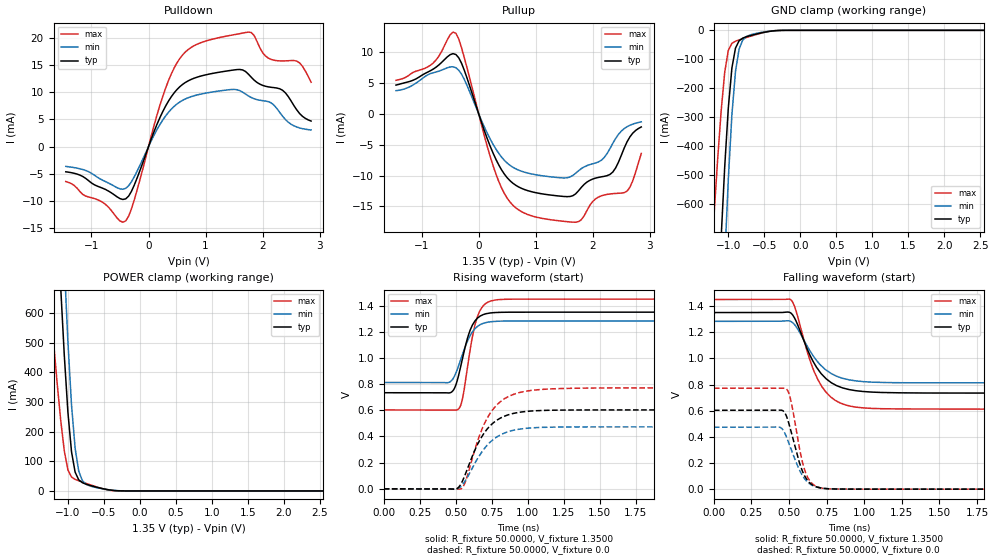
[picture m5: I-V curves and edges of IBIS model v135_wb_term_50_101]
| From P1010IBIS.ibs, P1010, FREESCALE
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[Model] v135_wb_term_50_101
|   Model v135_wb_term_50_101
| This model was characterised for following simulation conditions:
| External (pad) voltage:
|   - Typ: 1.35V,   - Min: 1.283V,   - Max: 1.45V
| Library cells for typ/min/max conditions are connected as defined below:
|  chip_pad - External Pad
|  ipp_do - Core Input
|  ipp_obe - Output Buffer Enable
|  esd_boost - vdd_io
|  gnd_io - gnd_io
|  vdd_d - vdd_d
|  vdd_io - vdd_io
|  vipp_dse_0 - gnd_io vdd_d gnd_io
|  vipp_dse_1 - vdd_d vdd_d gnd_io
|  vipp_dse_2 - vdd_d gnd_io gnd_io
|  vipp_dse_3 - gnd_io
|  vipp_dse_4 - gnd_io vdd_d gnd_io
|  vipp_dse_5 - vdd_d vdd_d gnd_io
|  vipp_dse_6 - vdd_d gnd_io vdd_d
|  vipp_dse_7 - gnd_io vdd_d gnd_io
|  vsel[0] - vdd_d
|  vsel[1] - gnd_io
|  vtermsel_0 - vdd_d
|  vtermsel_1 - gnd_io
|  vtermsel_2 - vdd_d
| All other pins connected to ground
Model_type I/O
Polarity   Non-Inverting
Enable   Active-High
Vinl =   0.5150V
Vinh =   0.9350V
Vmeas =  0.6750V
Cref =   0.0F
Rref =   50.0000
Vref =   0.6750V
C_comp   2.2026pF   1.9235pF   2.5884pF
[Receiver Thresholds]
Vth   =  0.675V
Vinh_ac  =  0.160V
Vinh_dc  =  0.090V
Vinl_ac  = -0.160V
Vinl_dc  = -0.090V
[Temperature Range]   65.0000   0.1250k   -40.0000
[Voltage Range]   1.3500V   1.2830V   1.4500V
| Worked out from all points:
|   slope of the pulldown table from 0 to 0.203 V, typ, clamps not added: 37.5 ohm
|   slope of the pullup table from 0 to 0.203 V, typ, clamps not added: 38.4 ohm
|   GND clamp passes 1 mA (typ) near -0.33 V on its own axis
|   POWER clamp passes 1 mA (typ) near -0.33 V on its own axis
|   rising waveform, R_fixture 50.0000, V_fixture 1.3500: 20-80 % time 87.9ps typ, 100ps min, 80.4ps max; typ from 0.734 V to 1.35 V
|   rising waveform, R_fixture 50.0000, V_fixture 0.0: 20-80 % time 169ps typ, 179ps min, 171ps max; typ from 0 V to 0.603 V
|   falling waveform, R_fixture 50.0000, V_fixture 1.3500: 20-80 % time 167ps typ, 176ps min, 157ps max; typ from 1.35 V to 0.734 V
|   falling waveform, R_fixture 50.0000, V_fixture 0.0: 20-80 % time 91.9ps typ, 104ps min, 79.1ps max; typ from 0.603 V to 0 V
[Pulldown]
|Voltage   I(typ)   I(min)   I(max)
-1.45V    -4.625mA   -3.634mA   -6.414mA
-400mV    -9.605mA   -7.673mA   -13.66mA
-250mV    -7.089mA   -5.553mA   -9.807mA
350mV     8.383mA    6.321mA    12.15mA
600mV     11.48mA    8.545mA    16.91mA
900mV     12.94mA    9.633mA    19.06mA
1.6V      14.2mA     10.31mA    20.8mA
1.8V      12.79mA    9.052mA    21.01mA
2.05V     11.12mA    8.394mA    16.69mA
2.35V     10.38mA    5.608mA    15.77mA
2.6V      6.75mA     3.61mA     15.74mA
2.85V     4.71mA     3.07mA     11.85mA
[Pullup]
|Voltage   I(typ)   I(min)   I(max)
-1.45V    4.66mA     3.76mA     5.44mA
-850mV    6.973mA    6.515mA    7.855mA
-400mV    9.617mA    7.475mA    13.06mA
350mV     -8.259mA   -6.386mA   -10.92mA
600mV     -11.25mA   -8.661mA   -14.82mA
950mV     -12.67mA   -9.781mA   -16.59mA
1.55V     -13.42mA   -10.36mA   -17.47mA
1.75V     -12.46mA   -9.22mA    -17.46mA
2.05V     -10.41mA   -7.958mA   -13.77mA
2.35V     -9.439mA   -4.799mA   -12.94mA
2.6V      -4.545mA   -2.088mA   -12.52mA
2.85V     -2.121mA   -1.298mA   -6.418mA
[GND_clamp]
|Voltage   I(typ)   I(min)   I(max)
-1.45V    -2.871A    -3.678A    -1.723A
-1.25V    -1.593A    -2.178A    -850.1mA
-1.2V     -1.288A    -1.811A    -645.5mA
-1.1V     -719.6mA   -1.112A    -280.3mA
-1.05V    -471.8mA   -794.7mA   -144.9mA
-1V       -268.3mA   -514.7mA   -69.38mA
-950mV    -129.9mA   -291mA     -44.9mA
-900mV    -61.27mA   -141.6mA   -37.53mA
-850mV    -36.06mA   -64.84mA   -33.07mA
-700mV    -18.64mA   -16.18mA   -21.16mA
-300mV    -565.4uA   -490.6uA   -354.2uA
2.85V     0A         0A         0A
[POWER_clamp]
|Voltage   I(typ)   I(min)   I(max)
-1.4V     2.365A     3.105A     1.115A
-1.25V    1.489A     2.054A     650.9mA
-1.15V    939.9mA    1.38A      364.8mA
-1.1V     686mA      1.062A     238.2mA
-1.05V    456.3mA    765.7mA    134.7mA
-1V       265.4mA    502.8mA    70.73mA
-950mV    132.2mA    289.8mA    46.77mA
-900mV    63.54mA    144.2mA    39.01mA
-850mV    37.51mA    67.07mA    34.23mA
-800mV    27.91mA    35.09mA    29.86mA
-450mV    4.485mA    4.459mA    3.638mA
2.9V      0A         0A         0A
[Ramp]
| variable   typ   min   max
dV/dt_r  0.3618/0.1692n   0.2841/0.1787n   0.4631/0.1710n
dV/dt_f  0.3693/0.1674n   0.2822/0.1757n   0.5055/0.1568n
R_load = 50.0000
[Rising Waveform]
R_fixture= 50.0000
V_fixture= 1.3500
V_fixture_min= 1.2830
V_fixture_max= 1.4500
|time   V(typ)   V(min)   V(max)
0s        734.4mV    812.7mV    602.8mV
457.8ps   733.2mV    815.7mV    602.8mV
518.2ps   857mV      934.1mV    608.8mV
545.7ps   989mV      1.023V     680.3mV
588.8ps   1.176V     1.146V     980.2mV
624.6ps   1.267V     1.212V     1.209V
651ps     1.304V     1.241V     1.316V
695.4ps   1.333V     1.266V     1.403V
766.3ps   1.347V     1.279V     1.441V
5ns       1.35V      1.283V     1.45V
[Rising Waveform]
R_fixture= 50.0000
V_fixture= 0.0
V_fixture_min= 0.0
V_fixture_max= 0.0
|time   V(typ)   V(min)   V(max)
0s        6.631uV    37.82uV    88.43nV
490ps     -2.257mV   -2.269mV   47.56uV
539.5ps   42.92mV    21.66mV    2.357mV
570.9ps   122.5mV    68.82mV    65.23mV
650ps     336.3mV    227.4mV    359.3mV
695.5ps   423.5mV    302.6mV    489.1mV
745.8ps   489.1mV    363.2mV    587.8mV
856.7ps   562.6mV    434.3mV    700mV
1.022ns   594.5mV    465.4mV    751.9mV
5ns       603mV      473.6mV    771.8mV
[Falling Waveform]
R_fixture= 50.0000
V_fixture= 1.3500
V_fixture_min= 1.2830
V_fixture_max= 1.4500
|time   V(typ)   V(min)   V(max)
0s        1.35V      1.283V     1.45V
510.3ps   1.347V     1.282V     1.449V
544.5ps   1.29V      1.246V     1.369V
613.7ps   1.09V      1.107V     1.078V
646.6ps   1.006V     1.043V     959.4mV
719.1ps   876.2mV    938mV      782.2mV
805.7ps   797.9mV    869.1mV    679.9mV
943.3ps   752.7mV    827.7mV    627.2mV
1.408ns   735mV      812.8mV    612.6mV
5ns       734.4mV    812.7mV    607.5mV
[Falling Waveform]
R_fixture= 50.0000
V_fixture= 0.0
V_fixture_min= 0.0
V_fixture_max= 0.0
|time   V(typ)   V(min)   V(max)
0s        603mV      473.6mV    771.8mV
433.7ps   603.9mV    474.7mV    771.7mV
460.6ps   598.5mV    451.4mV    772.3mV
484.1ps   553.9mV    395mV      763.2mV
510.7ps   452.1mV    313.2mV    683.6mV
574.5ps   182.6mV    133.7mV    281.1mV
608.4ps   91.9mV     72.41mV    131.1mV
653.5ps   33.35mV    29.03mV    42.48mV
729.3ps   6.051mV    6.156mV    6.211mV
5ns       6.793uV    38.19uV    132.9nV
